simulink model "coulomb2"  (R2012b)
settings: Solver=ode45  StartTime=0.0  StopTime=10.0  RelTol=1e-3
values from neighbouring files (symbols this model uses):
  c = 2200    [coulomb_1.m]    (also in coulomb_10.m = 0.1; coulomb_11.m = 0; coulomb_2.m; coulomb_3.m)
  Fex_ampl = 800    [coulomb_1.m]    (also in coulomb_2.m; coulomb_3.m; coulomb_4.m; coulomb_5.m)
  fu = 0.02    [coulomb_1.m]    (also in coulomb_2.m; coulomb_3.m; coulomb_4.m; coulomb_5.m = 0.1)
  m = 400    [coulomb_1.m]    (also in coulomb_10.m = 10; coulomb_11.m = 10; coulomb_2.m; coulomb_3.m)
  v0 = 0    [coulomb_1.m]    (also in coulomb_2.m; coulomb_3.m; coulomb_4.m; coulomb_5.m)
  y0 = 0    [coulomb_1.m]    (also in coulomb_2.m; coulomb_3.m; coulomb_4.m; coulomb_5.m)

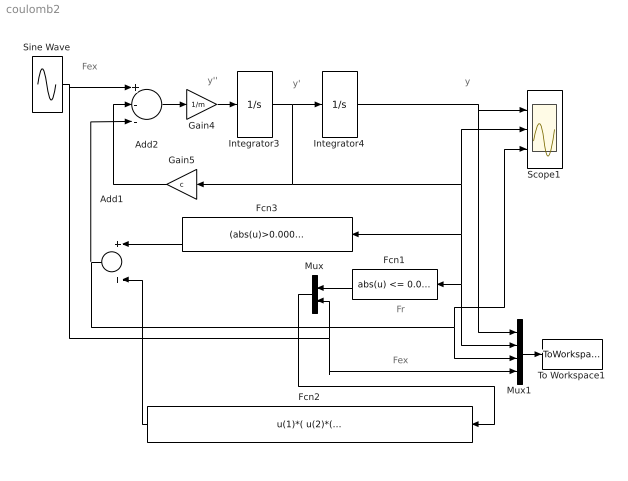
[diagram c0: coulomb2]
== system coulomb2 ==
  note: Fex
  note: Fr
  note: Fex
  note: y
  note: y'
  note: y''
  Add1 : Sum
  Add2 : Sum  Inputs=+--
  Fcn1 : Fcn  Expr=abs(u) <= 0.0001
  Fcn2 : Fcn  Expr=u(1)*( u(2)*(FG >abs(u(2)))+FG*sgn(u(2))*(abs(u(2))>=FG))
  Fcn3 : Fcn  Expr=(abs(u)>0.0001)*(FG*sgn(u))
  Gain4 : Gain  Gain=1/m
  Gain5 : Gain  Gain=c
  Integrator3 : Integrator  InitialCondition=v0
  Integrator4 : Integrator  InitialCondition=y0
  Mux : Mux  Inputs=2
  Mux1 : Mux
  Scope1 : Scope  NumInputPorts=3
  Sine Wave : Sin  Amplitude=Fex_ampl  Frequency=2*pi*fu  SampleTime=0
  To Workspace1 : ToWorkspace  VariableName=y  SampleTime=-1  SaveFormat=Structure With Time
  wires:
  Add2/1 -> Gain4/1
  Gain4/1 -> Integrator3/1
  Gain5/1 -> Add2/2
  Integrator4/1 -> Mux1/1, Scope1/1
  Mux1/1 -> To Workspace1/1
  Sine Wave/1 -> Mux/2, Mux1/4, Add2/1
  Fcn3/1 -> Add1/1
  Integrator3/1 -> Mux1/2, Fcn1/1, Fcn3/1, Scope1/2, Gain5/1, Integrator4/1
  Fcn2/1 -> Add1/2
  Fcn1/1 -> Mux/1
  Mux/1 -> Fcn2/1
  Add1/1 -> Add2/3, Scope1/3, Mux1/3
